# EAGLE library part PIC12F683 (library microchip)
8-Pin Flash-Based, 8-Bit CMOS Microcontrollers with nanoWatt Technology Source: http://ww1.microchip.com/downloads/en/DeviceDoc/41211D_.pdf
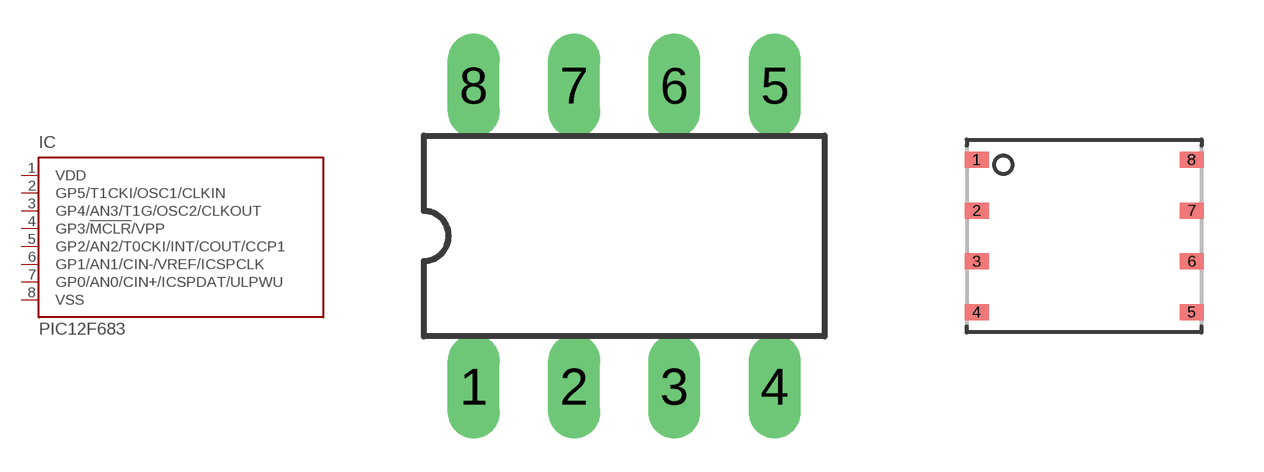
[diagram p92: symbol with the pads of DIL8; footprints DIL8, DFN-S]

Designator prefix IC

## PIC12F683P (MF: MICROCHIP; MPN: PIC12F683-I/P; OC_FARNELL: 9759034; OC_NEWARK: 89H0442)  [DIL8]
1  VDD  pwr
2  GP5/T1CKI/OSC1/CLKIN
3  GP4/AN3/T1G/OSC2/CLKOUT
4  GP3/!MCLR!/VPP
5  GP2/AN2/T0CKI/INT/COUT/CCP1
6  GP1/AN1/CIN-/VREF/ICSPCLK
7  GP0/AN0/CIN+/ICSPDAT/ULPWU
8  VSS  pwr

## PIC12F683DS (MF: MICROCHIP; MPN: PIC12F683-I/MF; OC_FARNELL: 1137331; OC_NEWARK: 89H0441)  [DFN-S]
Pads as for DIL8

## PIC12F683SN (MF: MICROCHIP; MPN: PIC12F683-I/SN; OC_FARNELL: 9759042; OC_NEWARK: 61K3434)  [SO-08]
Pads as for DIL8

## PIC12F683MD (MF: MICROCHIP; MPN: PIC12F683-I/MD; OC_FARNELL: 4057368; OC_NEWARK: 56K7230)  [DFN8-4X4]
Pads as for DIL8

## Footprint DIL8 (pad centres in mm)
Dual In Line package type P
drill 0.813 long: 1 -3.81,-3.81; 2 -1.27,-3.81; 3 1.27,-3.81; 4 3.81,-3.81; 5 3.81,3.81; 6 1.27,3.81; 7 -1.27,3.81; 8 -3.81,3.81

## Footprint DFN-S (pad centres in mm)
8-Lead Plastic Dual Flat No Lead Package (MF) 6x5 mm Body (DFN-S) Source: http://www.microchip.com .. 41190c.pdf
smd 0.6 x 0.4: 1 -2.69,1.905; 2 -2.69,0.635; 3 -2.69,-0.635; 4 -2.69,-1.905; 5 2.69,-1.905; 6 2.69,-0.635; 7 2.69,0.635; 8 2.69,1.905

## Footprint SO-08 (pad centres in mm)
Small Outline Narrow Plastic Gull Wing 150-mil body, package type SN
smd 0.6 x 2.2: 1 -1.905,-2.6; 2 -0.635,-2.6; 3 0.635,-2.6; 4 1.905,-2.6; 5 1.905,2.6; 6 0.635,2.6; 7 -0.635,2.6; 8 -1.905,2.6

## Footprint DFN8-4X4 (pad centres in mm)
8-Lead Plastic Dual Flat, No Lead Package (MD) 4x4x0.9 mm Body [DFN] Source: http://ww1.microchip.com/downloads/en/DeviceDoc/41211D_.pdf
smd 0.8 x 0.4: 1 -1.65,1.2; 2 -1.65,0.4; 3 -1.65,-0.4; 4 -1.65,-1.2; 5 1.65,-1.2; 6 1.65,-0.4; 7 1.65,0.4; 8 1.65,1.2
smd 2.2 x 3: EXP 0,0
